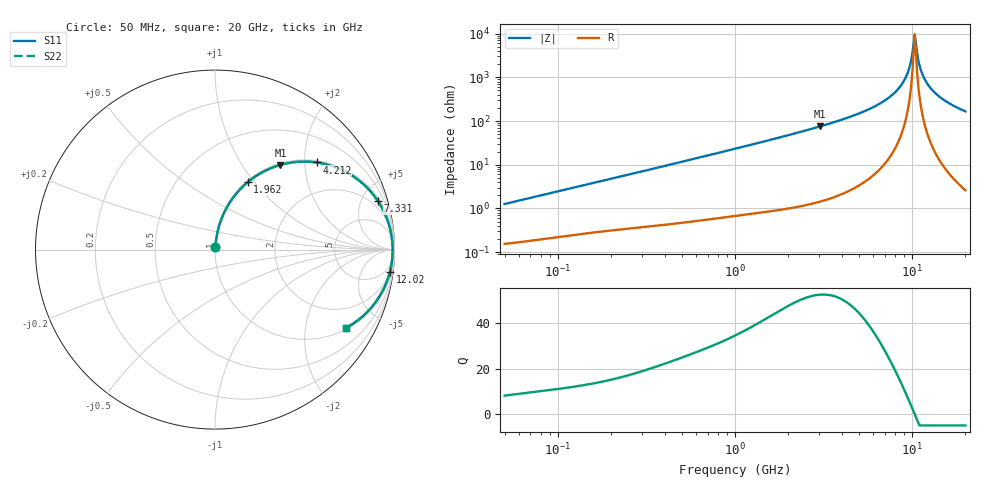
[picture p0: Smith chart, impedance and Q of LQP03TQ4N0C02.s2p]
!Murata Part Number: LQP03TQ4N0C02
!These Parameters are Measured in Series Mode Connection
!  o--[Z]--o
!Port1  Port2
!  o-------o
!Freq. Start=50[MHz] Stop=20[GHz], 401[Steps]
# Hz S RI R 50
!Freq.(Hz) S11(Real) S11(Imag) S21(Real) S21(Imag) S12(Real) S12(Imag) S22(Real) S22(Imag)
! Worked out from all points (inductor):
!   401 points, 50 MHz to 20 GHz, reference 50 ohm
!   read as one part in series: L = 3.95 nH near 51.52 MHz
!   highest Q = 52.7 at 3.03 GHz (marker M1), where L = 3.96 nH
!   self-resonance near 10.35 GHz
!   S11 on the Smith chart (normalised r, x): 50 MHz: 1.00, +0.03; 1.962 GHz: 1.02, +0.93; 4.212 GHz: 1.05, +2.29; 7.331 GHz: 1.26, +6.67; 12.02 GHz: 2, -16; 20 GHz: 1.05, -3.32
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5e7  0.00169 0.0125  0.9983 -0.0125  0.9983 -0.0125  0.00169 0.0125
1.364002e8  0.00366 0.0326  0.9963 -0.0326  0.9963 -0.0326  0.00366 0.0326
3.721004e8  0.0115 0.0856  0.9885 -0.0856  0.9885 -0.0856  0.0115 0.0856
1e9  0.0566 0.2171  0.9434 -0.2171  0.9434 -0.2171  0.0566 0.2171
1.962148e9  0.1823 0.3757  0.8177 -0.3757  0.8177 -0.3757  0.1823 0.3757
2.728004e9  0.3113 0.4535  0.6887 -0.4535  0.6887 -0.4535  0.3113 0.4535
3.029571e9  0.3647 0.472  0.6353 -0.472  0.6353 -0.472  0.3647 0.472
4.212059e9  0.5669 0.4855  0.4331 -0.4855  0.4331 -0.4855  0.5669 0.4855
5.769027e9  0.7772 0.4034  0.2228 -0.4034  0.2228 -0.4034  0.7772 0.4034
7.331367e9  0.9087 0.2688  0.0913 -0.2688  0.0913 -0.2688  0.9087 0.2688
7.442007e9  0.9153 0.2586  0.0847 -0.2586  0.0847 -0.2586  0.9153 0.2586
8.389408e9  0.9585 0.1708  0.0415 -0.1708  0.0415 -0.1708  0.9585 0.1708
9.178299e9  0.9792 0.0994  0.0208 -0.0994  0.0208 -0.0994  0.9792 0.0994
9.600142e9  0.9854 0.0626  0.0146 -0.0626  0.0146 -0.0626  0.9854 0.0626
1.004137e10  0.9889 0.0254  0.0111 -0.0254  0.0111 -0.0254  0.9889 0.0254
1.034674e10  0.9897 0.000464  0.0103 -0.000464  0.0103 -0.000464  0.9897 0.000464
1.066139e10  0.9891 -0.0245  0.0109 0.0245  0.0109 0.0245  0.9891 -0.0245
1.115139e10  0.986 -0.0618  0.014 0.0618  0.014 0.0618  0.986 -0.0618
1.201863e10  0.9745 -0.1229  0.0255 0.1229  0.0255 0.1229  0.9745 -0.1229
1.314879e10  0.9509 -0.1933  0.0491 0.1933  0.0491 0.1933  0.9509 -0.1933
1.460232e10  0.9108 -0.2692  0.0892 0.2692  0.0892 0.2692  0.9108 -0.2692
2e10  0.731 -0.4357  0.269 0.4357  0.269 0.4357  0.731 -0.4357
